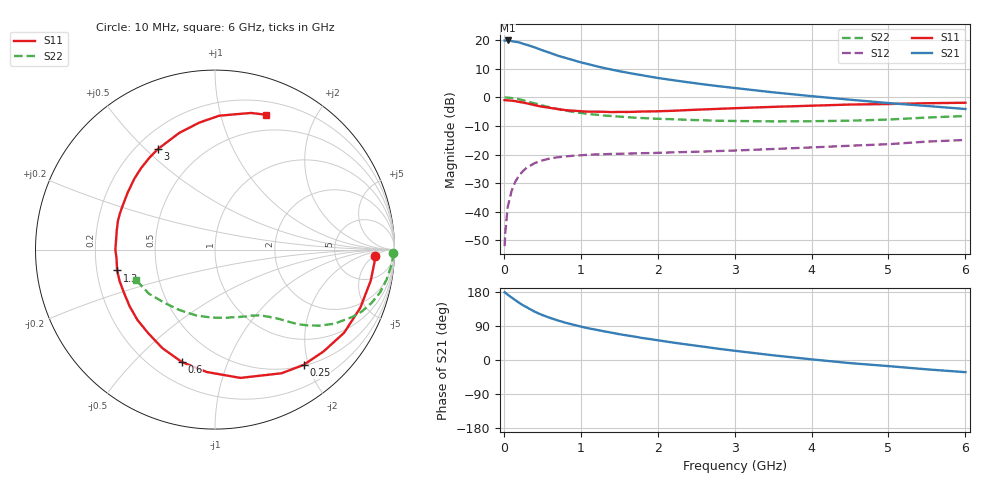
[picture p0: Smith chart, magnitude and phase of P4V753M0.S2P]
! SIEMENS Small Signal Semiconductors
! BFP182
! Si NPN RF Bipolar Junction Transistor in SOT143
! VCE = 0.75 V  IC = 3 mA
! Common Emitter S-Parameters:  March  1996
# GHz  S  MA  R  50
!  f  S11  S21  S12  S22
! GHz  MAG  ANG  MAG  ANG  MAG  ANG  MAG  ANG
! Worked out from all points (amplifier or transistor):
!   36 points, 10 MHz to 6 GHz, reference 50 ohm
!   highest |S21| = 19.9 dB at 50 MHz (marker M1)
!   |S21| within 3 dB of that: start of sweep to 458.6 MHz
!   unconditionally stable (mu >= 1): 1.804 GHz to end of sweep
!   at 250 MHz: K = 0.16, MSG = 22.2 dB, |S12| = -25.8 dB
!   at 1.4 GHz: K = 0.83, MSG = 14.7 dB, |S12| = -19.8 dB
!   at 6 GHz: K = 1.12, MAG = 3.3 dB, |S12| = -14.9 dB
!   S11 on the Smith chart (normalised r, x): 10 MHz: 16, -5; 250 MHz: 0.51, -1.92; 600 MHz: 0.32, -0.70; 1.3 GHz: 0.29, -0.10; 3 GHz: 0.29, +0.55; 6 GHz: 0.33, +1.39
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0.01  0.8916 -2.2  9.76 178.8  0.0025 84.7  0.9912 -1.0
0.02  0.8917 -4.4  9.787 177.6  0.0045 84.4  0.9931 -2.0
0.05  0.8848 -11.3  9.843 172.4  0.012 87.2  0.9869 -5.0
0.15  0.8556 -32.8  9.35 157.8  0.0337 71.4  0.9499 -14.6
0.2  0.8292 -43.2  9.088 150.8  0.0433 66.7  0.9208 -18.9
0.25  0.81 -52.5  8.612 144.4  0.0515 61.5  0.8873 -22.9
0.3  0.7824 -61.7  8.255 138.9  0.0591 56.9  0.8526 -26.1
0.4  0.7288 -78.8  7.462 127.6  0.0706 48.9  0.7833 -31.8
0.5  0.6836 -93.8  6.639 118.6  0.0788 42.5  0.7192 -36.1
0.6  0.6532 -106.4  5.975 111.2  0.0853 37.8  0.6666 -39.3
0.7  0.6224 -118.1  5.341 104.5  0.0894 33.8  0.6246 -41.8
0.8  0.5961 -128.6  4.884 98.5  0.0925 30.7  0.5873 -43.7
0.9  0.5835 -137.7  4.468 93.3  0.0952 27.9  0.5565 -45.4
1.1  0.5611 -154.9  3.789 83.6  0.0989 24.3  0.5116 -48.4
1.3  0.5577 -168.0  3.255 75.8  0.101 21.5  0.4808 -51.1
1.8  0.5638 163.7  2.423 58.1  0.1055 18.5  0.4337 -57.8
2.2  0.5812 146.8  1.99 46.0  0.109 16.9  0.4136 -64.3
3  0.6443 119.6  1.454 24.4  0.1173 15.9  0.3853 -80.6
3.5  0.6801 107.0  1.221 12.4  0.1248 15.3  0.3793 -92.7
4.5  0.7464 88.2  0.907 -8.2  0.1423 13.4  0.3899 -119.9
5.5  0.7874 75.2  0.705 -24.7  0.168 10.3  0.4426 -146.3
6  0.803 69.4  0.624 -32.1  0.1796 6.8  0.4709 -158.7
